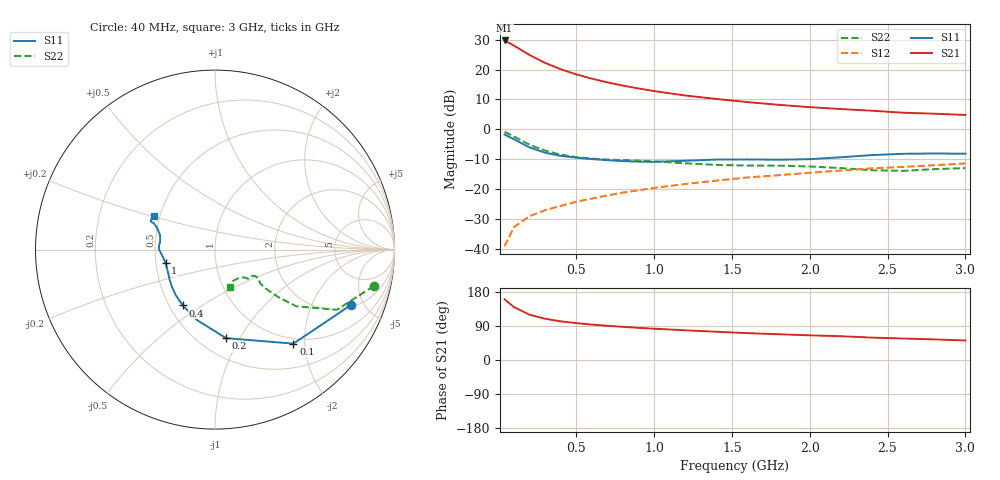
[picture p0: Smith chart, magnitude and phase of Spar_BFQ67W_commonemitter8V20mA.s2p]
! Filename:  BFQ67WK.S2P  Version:  4.0
! NXP part #: BFQ67W  Date: Jun 1994
! Bias condition: Vce=8V, Ic=20mA
#  MHz  S  MA  R  50
! Freq  S11  S21  S12  S22
!GUM [dB]
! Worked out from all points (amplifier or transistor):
!   21 points, 40 MHz to 3 GHz, reference 50 ohm
!   highest |S21| = 29.8 dB at 40 MHz (marker M1)
!   |S21| within 3 dB of that: start of sweep to 140.5 MHz
!   unconditionally stable (mu >= 1): 673.9 MHz to end of sweep
!   at 300 MHz: K = 0.76, MSG = 24.7 dB, |S12| = -27.1 dB
!   at 1 GHz: K = 1.07, MAG = 14.6 dB, |S12| = -19.7 dB
!   at 3 GHz: K = 1.03, MAG = 7.1 dB, |S12| = -11.4 dB
!   lowest NFmin = 2.30 dB at 1 GHz
!   S11 on the Smith chart (normalised r, x): 40 MHz: 2.14, -3.98; 100 MHz: 0.90, -1.77; 200 MHz: 0.67, -0.88; 400 MHz: 0.59, -0.42; 1 GHz: 0.56, -0.09; 3 GHz: 0.46, +0.20
40  0.817 -22.3  30.84 160.0  0.011 78.5  0.908 -12.9
100  0.682 -50.2  25.28 139.7  0.023 66.5  0.757 -26.3
200  0.497 -82.9  17.61 119.6  0.035 60.4  0.552 -34.9
300  0.405 -104.4  12.99 108.9  0.044 60.6  0.44 -36.9
400  0.359 -120.0  10.17 102.0  0.052 62.4  0.377 -37.4
500  0.335 -130.8  8.336 97.3  0.061 63.9  0.342 -37.4
600  0.317 -139.1  7.061 93.5  0.069 65.8  0.322 -37.1
700  0.304 -146.3  6.127 90.3  0.078 67.1  0.311 -36.6
800  0.293 -152.5  5.405 87.5  0.087 68.2  0.305 -35.6
900  0.287 -158.8  4.842 84.9  0.095 68.9  0.298 -34.6
1000  0.285 -164.7  4.373 82.6  0.104 69.5  0.29 -33.7
1200  0.297 -174.1  3.69 78.4  0.121 70.3  0.269 -33.2
1400  0.311 -179.7  3.226 74.6  0.138 70.9  0.253 -35.3
1600  0.313 176.3  2.858 70.9  0.156 70.4  0.247 -39.3
1800  0.309 171.9  2.573 68.0  0.17 70.7  0.246 -41.5
2000  0.316 165.4  2.351 65.1  0.187 70.9  0.238 -42.1
2200  0.34 160.1  2.187 62.8  0.204 71.2  0.224 -43.7
2400  0.37 156.7  2.048 59.1  0.222 70.7  0.206 -50.7
2600  0.389 156.5  1.897 56.7  0.234 70.0  0.201 -59.8
2800  0.393 155.3  1.827 54.4  0.25 70.2  0.215 -65.2
3000  0.39 151.3  1.74 51.4  0.268 69.8  0.224 -67.6
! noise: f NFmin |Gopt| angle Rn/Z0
1000  2.3  0.271  83  0.297
